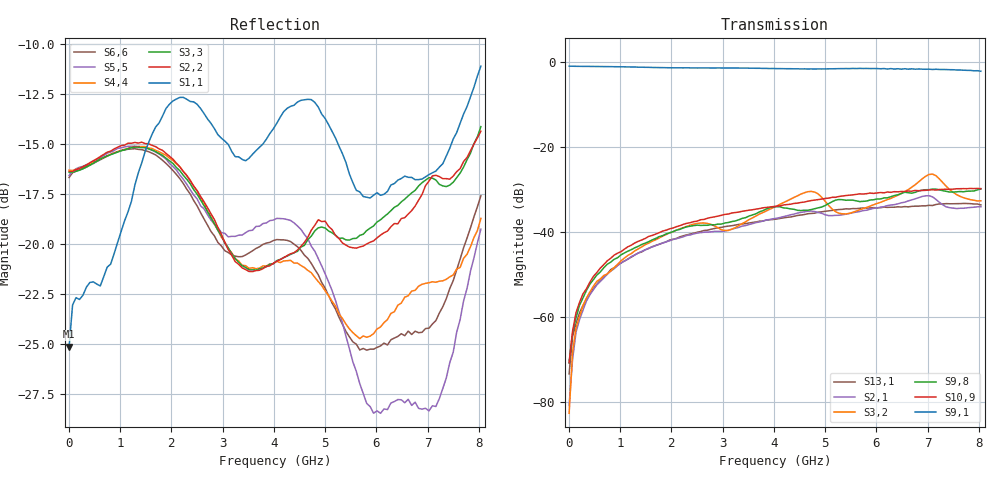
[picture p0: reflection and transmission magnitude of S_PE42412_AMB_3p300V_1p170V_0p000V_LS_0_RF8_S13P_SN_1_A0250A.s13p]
! Device ID: PE42412
! File Path: z:\PE42412\TE_GND_Post_Char_S-Param\All Parts\AMB\3p300\LS_0_RF8\PE42412_AMB_3p300V_1p170V_0p000V_LS_0_RF8_S13P_SN_1_A0250A.s13p
! Serial: 1
! Lot: A0250A
! Temp: AMB
! VDD: 3.300
! VSS: 0.000
! Control_Hi: 1.170
! Control_Lo: 0.000
! Logic State: LS_0_RF8
! Port 1:
! Port 2:
! Port 3:
! Port 4:
! Port 5:
! Port 6:
! Port 7:
! Port 8:
! Port 9:
! Port 10:
! Port 11:
! Port 12:
! Port 13:
! ThroughPath:1-9
! IDD: 0.0001077919
! ISS/IDD2: 9.05e-008
! IDMM3/IDD3: -1.546e-007
! Comment:
#  Hz  S  RI  R  50
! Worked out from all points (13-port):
!   120 points, 10 MHz to 8.037 GHz, reference 50 ohm
!   strongest paths, dB at 10 MHz, 2.034 GHz, 4.057 GHz, 6.08 GHz, 8.037 GHz:
!     S9,1: -1.0, -1.3, -1.5, -1.6, -2.2
!     S10,9: -70.8, -39.1, -33.9, -30.7, -29.8
!     S9,8: -70.8, -39.9, -34.1, -32.2, -29.9
!     S3,2: -82.7, -40.0, -33.9, -33.0, -32.7
!     S2,1: -80.8, -41.8, -36.8, -34.2, -34.1
!     S13,1: -73.4, -41.7, -37.0, -34.3, -33.6
!   lowest |S11| = -25.1 dB at 10 MHz (marker M1), VSWR 1.12, Z = 55.2 - j2.66 ohm
!   |S11| at or under -10 dB: start of sweep to end of sweep
